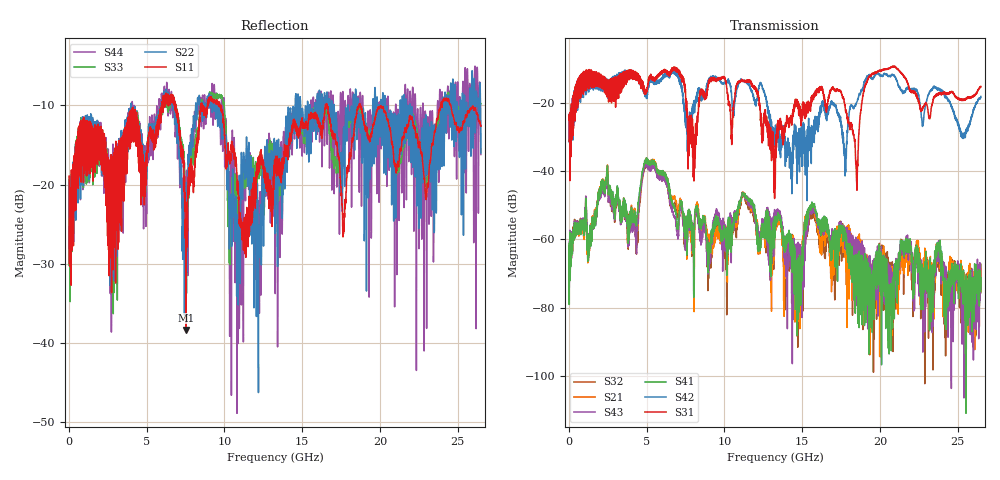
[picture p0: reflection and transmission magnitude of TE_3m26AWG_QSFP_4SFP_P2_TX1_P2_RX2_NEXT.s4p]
!Agilent Technologies,N5222A,MY51421691,A.10.00.00
!Agilent N5222A: A.10.00.00
!Date: Friday, January 30, 2015 12:35:26
!Correction: S11(Full 4 Port(1,2,3,4))
!S12(Full 4 Port(1,2,3,4))
!S13(Full 4 Port(1,2,3,4))
!S14(Full 4 Port(1,2,3,4))
!S21(Full 4 Port(1,2,3,4))
!S22(Full 4 Port(1,2,3,4))
!S23(Full 4 Port(1,2,3,4))
!S24(Full 4 Port(1,2,3,4))
!S31(Full 4 Port(1,2,3,4))
!S32(Full 4 Port(1,2,3,4))
!S33(Full 4 Port(1,2,3,4))
!S34(Full 4 Port(1,2,3,4))
!S41(Full 4 Port(1,2,3,4))
!S42(Full 4 Port(1,2,3,4))
!S43(Full 4 Port(1,2,3,4))
!S44(Full 4 Port(1,2,3,4))
!S4P File: Measurements: <S11,S12,S13,S14>,
!<S21,S22,S23,S24>,
!<S31,S32,S33,S34>,
!<S41,S42,S43,S44>:
# Hz S  dB  R 50.0
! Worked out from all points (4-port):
!   2650 points, 10 MHz to 26.5 GHz, reference 50 ohm
!   strongest paths, dB at 10 MHz, 6.63 GHz, 13.26 GHz, 19.88 GHz, 26.5 GHz:
!     S31: -25.0, -10.3, -36.2, -10.8, -15.2
!     S42: -24.8, -11.3, -30.4, -11.5, -18.2
!     S41: -61.1, -49.4, -54.0, -69.0, -75.2
!     S43: -73.2, -52.1, -52.9, -67.7, -74.6
!     S21: -76.5, -48.1, -56.7, -67.1, -68.7
!     S32: -66.9, -50.8, -56.1, -69.2, -67.3
!   lowest |S11| = -38.3 dB at 7.52 GHz (marker M1), VSWR 1.02, Z = 51.2 + j0.207 ohm
!   |S11| at or under -10 dB: start of sweep to 5.957 GHz; 9.72 GHz to 16.5 GHz (6.777 GHz wide, 51.7 % of centre); 18.73 GHz to 23.91 GHz (5.183 GHz wide, 24.3 % of centre)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
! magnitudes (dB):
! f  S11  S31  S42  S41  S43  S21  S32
! 10 MHz  -18.9  -25.0  -24.8  -61.1  -73.2  -76.5  -66.9
! 2.38 GHz  -16.3  -13.1  -12.8  -44.1  -45.1  -43.7  -44.7
! 7.52 GHz  -38.3  -19.8  -22.9  -53.7  -54.7  -54.3  -55.2
! 17.33 GHz  -16.6  -16.4  -23.8  -58.8  -62.4  -58.1  -62.8
! 18.49 GHz  -11.0  -41.7  -20.0  -67.1  -59.9  -60.1  -62.6
! 19.59 GHz  -12.3  -11.4  -12.5  -72.9  -80.1  -72.7  -99.0
! 26.5 GHz  -12.6  -15.2  -18.2  -75.2  -74.6  -68.7  -67.3
